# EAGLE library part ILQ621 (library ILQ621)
Vishay Optocoupler ILQ621 Quad DC Input Transistor Output, 16-Pin PDIP, Through Hole Source: Datasheet
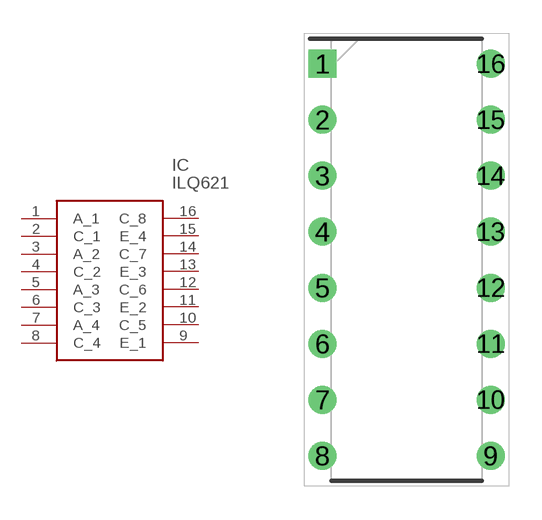
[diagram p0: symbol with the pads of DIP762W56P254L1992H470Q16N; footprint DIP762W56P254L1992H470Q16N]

Designator prefix IC

## ILQ621 (Description: Vishay Optocoupler ILQ621 Quad DC Input Transistor Output, 16-Pin PDIP, Through Hole; Height: 4.7mm; Manufacturer_Name: Vishay; Manufacturer_Part_Number: ILQ621; Mouser_Part_Number: 782-ILQ621; Mouser_Price-Stock: https://www.mouser.co.uk/ProductDetail/Vishay-Semiconductors/ILQ621?qs=xCMk%252BIHWTZMm5K87NCClyQ%3D%3D)  [DIP762W56P254L1992H470Q16N]
1  A_1
2  C_1
3  A_2
4  C_2
5  A_3
6  C_3
7  A_4
8  C_4
9  E_1
10  C_5
11  E_2
12  C_6
13  E_3
14  C_7
15  E_4
16  C_8

## Footprint DIP762W56P254L1992H470Q16N (pad centres in mm)
DIP-16
drill 0.76 pad 1.16 square: 1 -3.81,8.89
drill 0.76 pad 1.16: 2 -3.81,6.35; 3 -3.81,3.81; 4 -3.81,1.27; 5 -3.81,-1.27; 6 -3.81,-3.81; 7 -3.81,-6.35; 8 -3.81,-8.89; 9 3.81,-8.89; 10 3.81,-6.35; 11 3.81,-3.81; 12 3.81,-1.27; 13 3.81,1.27; 14 3.81,3.81; 15 3.81,6.35; 16 3.81,8.89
